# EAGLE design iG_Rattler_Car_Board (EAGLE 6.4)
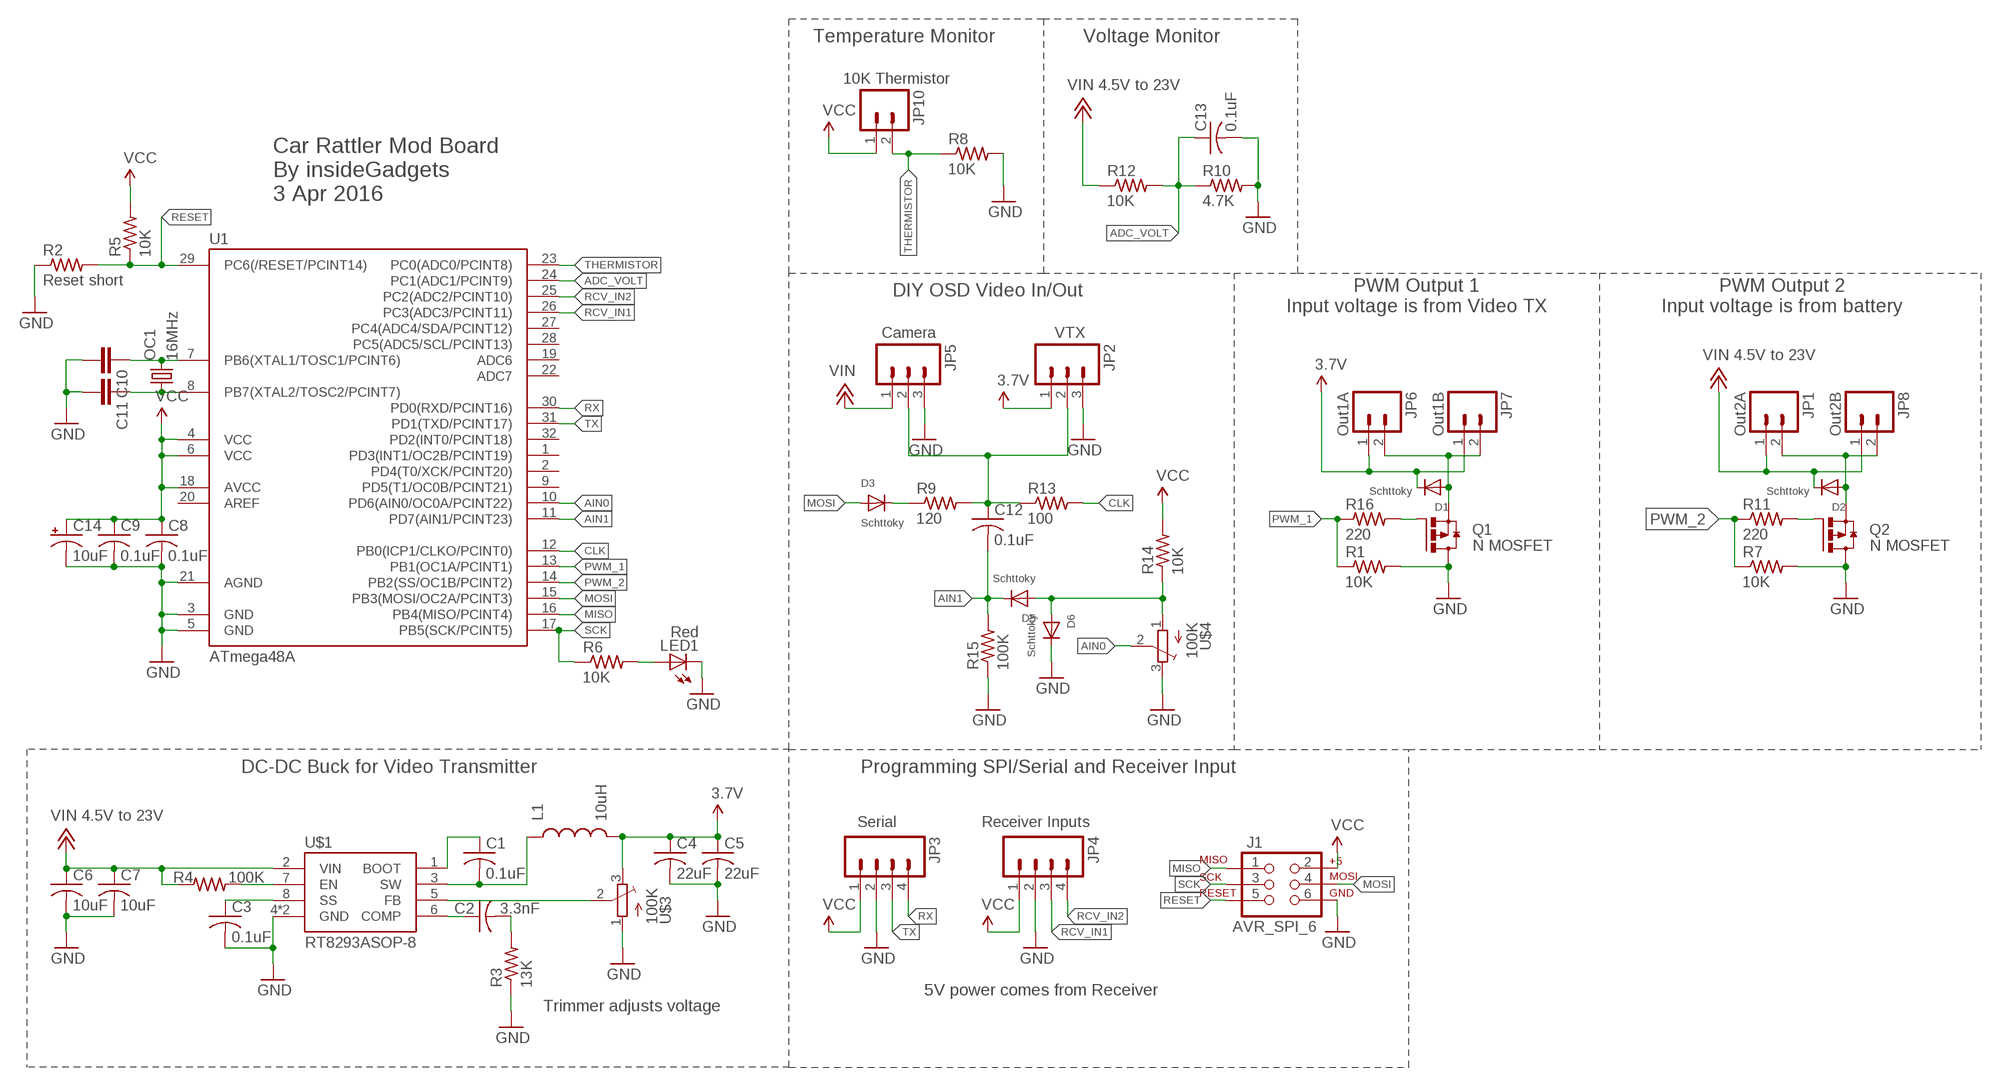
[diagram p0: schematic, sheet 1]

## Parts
C1  0.1uF  C-USC0603K  [C0603K]
C2  3.3nF  C-USC0603K  [C0603K]
C3  0.1uF  C-USC0603K  [C0603K]
C4  22uF  C-USC1206K  [C1206K]
C5  22uF  C-USC1206K  [C1206K]
C6  10uF  C-USC1206K  [C1206K]
C7  10uF  C-USC1206K  [C1206K]
C8  0.1uF  C-USC0805K  [C0805K]
C9  0.1uF  C-USC0805K  [C0805K]
C10  CAP0805  [0805]
C11  CAP0805  [0805]
C12  0.1uF  C-USC0805K  [C0805K]
C13  0.1uF  C-USC0805K  [C0805K]
C14  10uF  CPOL-US153CLV-0405  [153CLV-0405]
D1  Schttoky  DIODESOD-323  [SOD-323]
D2  Schttoky  DIODESOD-323  [SOD-323]
D3  Schttoky  DIODESOD-323  [SOD-323]
D5  Schttoky  DIODESOD-323  [SOD-323]
D6  Schttoky  DIODESOD-323  [SOD-323]
J1  AVR_SPI_6  AVR_SPI_PRG_6  [2X3_2]
JP1  Out2A  M02PTH  [1X02]
JP2  VTX  M03PTH  [1X03]
JP3  Serial  M04PTH  [1X04]
JP4  Receiver Inputs  M04PTH  [1X04]
JP5  Camera  M03PTH  [1X03]
JP6  Out1A  M02PTH  [1X02]
JP7  Out1B  M02PTH  [1X02]
JP8  Out2B  M02PTH  [1X02]
JP10  10K Thermistor  M02PTH  [1X02]
L1  10uH  INDUCTOR_7MM  [INDUCTOR7MM]
LED1  Red  LEDCHIP-LED0805-NS  [CHIP-LED0805-NS]
OC1  16MHz  XTAL-SMNOSILK  [XTAL32-25-NS]
Q1  N MOSFET  MOSFET_N_SMD_SOT23  [SUPER-SOT3]
Q2  N MOSFET  MOSFET_N_SMD_SOT23  [SUPER-SOT3]
R1  10K  R-US_R0805  [R0805]
R2  Reset short  R-US_R0805_2  [R0805_2]
R3  13K  R-US_R0603  [R0603]
R4  100K  R-US_R0603  [R0603]
R5  10K  R-US_R0805_2  [R0805_2]
R6  10K  R-US_R0805_2  [R0805_2]
R7  10K  R-US_R0805  [R0805]
R8  10K  R-US_R0805_2  [R0805_2]
R9  120  R-US_R0805_2  [R0805_2]
R10  4.7K  R-US_R0805_2  [R0805_2]
R11  220  R-US_R0805  [R0805]
R12  10K  R-US_R0805_2  [R0805_2]
R13  100  R-US_R0805_2  [R0805_2]
R14  10K  R-US_R0805_2  [R0805_2]
R15  100K  R-US_R0805_2  [R0805_2]
R16  220  R-US_R0805  [R0805]
U1  ATmega48A  MEGA48/88/168-AU  [TQFP32-08]
U$1  RT8293ASOP-8  [SOP-8]
U$3  100K  TRIMPOTTC33X  [TC33X]
U$4  100K  TRIMPOTTC33X  [TC33X]

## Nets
3.7V: C4.1 C5.1 D1.C JP2.1 JP6.1 JP7.1 L1.2 U$3.3(E)
5V: C8.1 C9.1 C14.+ J1.2 JP3.1 JP4.1 JP10.1 R5.2 R14.2 U1.4(VCC) U1.6(VCC) U1.18(AVCC) ; supply symbol labelled VCC
+12V: C6.1 C7.1 D2.C JP1.1 JP5.1 JP8.1 R4.1 R12.1 U$1.2(VIN) ; supply symbol labelled VIN 4.5V to 23V, VIN
ADC_VOLT: C13.1 R10.1 R12.2 U1.24(PC1(ADC1/PCINT9))
AIN0: U1.10(PD6(AIN0/OC0A/PCINT22)) U$4.2(S)
AIN1: C12.2 D5.C R15.2 U1.11(PD7(AIN1/PCINT23))
BOOT: C1.1 U$1.1(BOOT)
CLK: R13.2 U1.12(PB0(ICP1/CLKO/PCINT0))
COMP: C2.1 U$1.6(COMP)
EN: R4.2 U$1.7(EN)
FB: U$1.5(FB) U$3.2(S)
GND: C3.2 C4.2 C5.2 C6.2 C7.2 C8.2 C9.2 C10.2 C11.2 C13.2 C14.- D6.C J1.6 JP2.3 JP3.2 JP4.2 JP5.3 LED1.C Q1.2(D) Q2.2(D) R1.2 R2.1 R3.1 R7.2 R8.2 R10.2 R15.1 U1.3(GND) U1.5(GND) U1.21(AGND) U$1.4(GND) U$1.9(GND) U$3.1(A) U$4.3(E)
MISO: J1.1 U1.16(PB4(MISO/PCINT4))
MOSI: D3.A J1.4 U1.15(PB3(MOSI/OC2A/PCINT3))
N$1: C2.2 R3.2
N$3: D1.A JP6.2 JP7.2 Q1.3(S)
N$8: Q1.1(G) R16.2
N$10: LED1.A R6.2
N$13: D3.C R9.1
N$14: C11.1 OC1.1 U1.8(PB7(XTAL2/TOSC2/PCINT7))
N$15: C10.1 OC1.2 U1.7(PB6(XTAL1/TOSC1/PCINT6))
N$18: D5.A D6.A R14.1 U$4.1(A)
N$22: D2.A JP1.2 JP8.2 Q2.3(S)
N$27: Q2.1(G) R11.2
PWM_1: R1.1 R16.1 U1.13(PB1(OC1A/PCINT1))
PWM_2: R7.1 R11.1 U1.14(PB2(SS/OC1B/PCINT2))
RCV_IN1: JP4.3 U1.26(PC3(ADC3/PCINT11))
RCV_IN2: JP4.4 U1.25(PC2(ADC2/PCINT10))
RESET: J1.5 R2.2 R5.1 U1.29(PC6(/RESET/PCINT14))
RX: JP3.4 U1.30(PD0(RXD/PCINT16))
SCK: J1.3 R6.1 U1.17(PB5(SCK/PCINT5))
SS: C3.1 U$1.8(SS)
SW: C1.2 L1.1 U$1.3(SW)
THERMISTOR: JP10.2 R8.1 U1.23(PC0(ADC0/PCINT8))
TX: JP3.3 U1.31(PD1(TXD/PCINT17))
VIDEO: C12.1 JP2.2 JP5.2 R9.2 R13.1
Unconnected: U1.1(PD3(INT1/OC2B/PCINT19)) U1.2(PD4(T0/XCK/PCINT20)) U1.9(PD5(T1/OC0B/PCINT21)) U1.19(ADC6) U1.20(AREF) U1.22(ADC7) U1.27(PC4(ADC4/SDA/PCINT12)) U1.28(PC5(ADC5/SCL/PCINT13)) U1.32(PD2(INT0/PCINT18))

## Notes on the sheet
- Temperature Monitor | Voltage Monitor
- Car Rattler Mod Board
  By insideGadgets
  3 Apr 2016
- DIY OSD Video In/Out
- PWM Output 1
  Input voltage is from Video TX
- PWM Output 2
  Input voltage is from battery
- DC-DC Buck for Video Transmitter | Programming SPI/Serial and Receiver Input
- 5V power comes from Receiver
- Trimmer adjusts voltage

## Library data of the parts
C1-C9 C12 C13 = adafruit:C-US: CAPACITOR, American symbol
C10 C11 = SparkFun:CAP: Capacitor
C14 = rcl:CPOL-US: POLARIZED CAPACITOR, American symbol
D1-D3 D5 D6 = adafruit:DIODE: Diode
J1 = SparkFun:AVR_SPI_PRG_6: AVR ISP 6 Pin This is the reduced ISP connector for AVR programming. Common on Arduino. This footprint will take up less PCB space and can be used with a 10-pin to 6-pin adapter such as SKU: BOB-08508
JP1 JP6-JP8 JP10 = SparkFun:M02: Header 2
JP2 JP5 = SparkFun:M03: Header 3 Standard 3-pin 0.1" header. Use with straight break away headers (SKU : PRT-00116), right angle break away headers (PRT-00553), swiss pins (PRT-00743), machine pins (PRT-00117), and female headers (PRT-00115). Molex polarized connector foot print use with SKU : PRT-08232 with associated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
JP3 JP4 = SparkFun:M04: Header 4 Standard 4-pin 0.1" header. Use with straight break away headers (SKU : PRT-00116), right angle break away headers (PRT-00553), swiss pins (PRT-00743), machine pins (PRT-00117), and female headers (PRT-00115). Molex polarized connector foot print use with SKU : PRT-08231 with associated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
L1 = SparkFun:INDUCTOR_7MM
LED1 = adafruit:LED: LED
OC1 = adafruit:XTAL-SM
Q1 Q2 = transistor-power:MOSFET_N_SMD_SOT23
R1-R16 = adafruit:R-US_: RESISTOR, American symbol
U1 = avr-5:MEGA48/88/168
U$1 = alex:RT8293A
U$3 U$4 = adafruit:TRIMPOT: SMT trimmer potentiometer part number TC33X http://www.ladyada.net/library/eagle

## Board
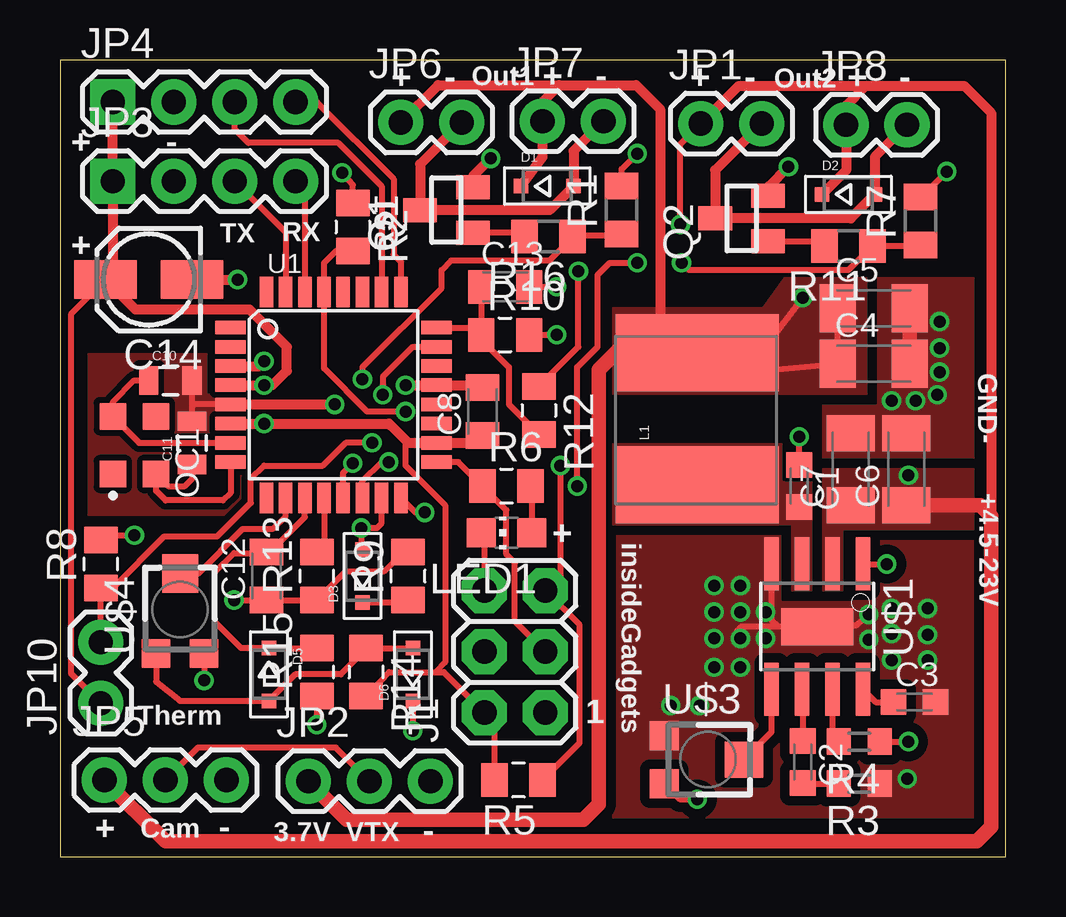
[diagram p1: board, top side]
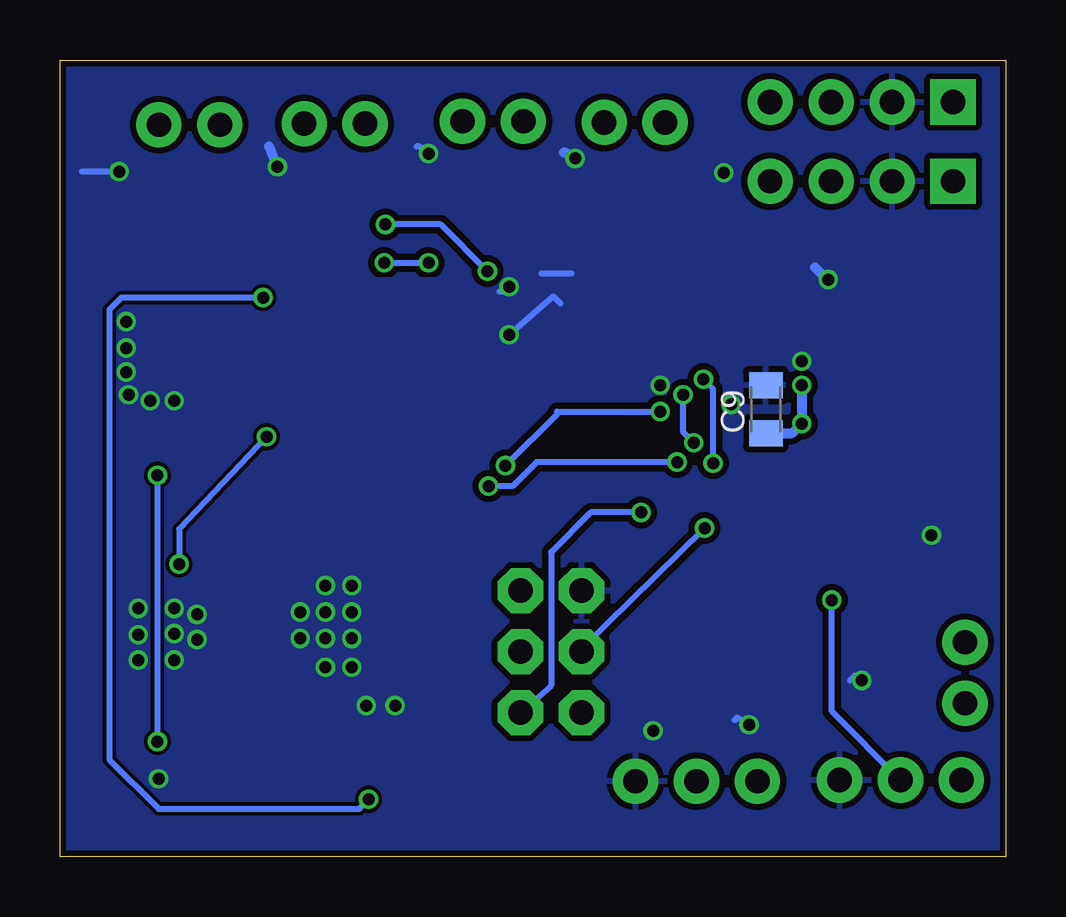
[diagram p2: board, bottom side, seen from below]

Size 39.4 x 33.2 mm. Coordinates in mm from the lower left corner, seen from the top.
Outline: 39.4,33.2 0,33.2 0,0 39.4,0 39.4,33.2
Copper layers (1*16): Top 0.035mm / dielectric 1.5mm / Bottom 0.035mm
Design rules "ITead_rule": minimum track width 6mil, minimum drill 12mil, track to track 6mil, track to pad 6mil, pad to pad 6mil, via to via 6mil, smd to smd 0mil, copper to edge 10mil, drill to drill 10mil, minimum pad ring 10mil, minimum via ring 6mil, stop-mask expansion 2mil, vias tented up to drill 100mil, thermal gap 10mil

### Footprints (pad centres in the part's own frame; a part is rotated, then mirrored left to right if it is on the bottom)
C0603K = smd 1.05 x 1.08: 1 -0.875,0; 2 0.875,0
C1206K = smd 1.5 x 2: 1 -1.5,0; 2 1.5,0
C0805K = smd 1.1 x 1.4: 1 -1,0; 2 1,0
0805 = smd 0.8 x 1.2: 1 -0.9,0; 2 0.9,0
153CLV-0405 = smd 2.6 x 1.6: + 1.8,0; - -1.8,0
SOD-323 = smd 0.6 x 0.6: A 1.1,0; C -1.1,0
2X3_2 = drill 1.016 pad 1.88 octagon: 1 -2.54,-1.27; 2 -2.54,1.27; 3 0,-1.27; 4 0,1.27; 5 2.54,-1.27; 6 2.54,1.27
1X02 = drill 1.016 pad 1.88: 1 0,0; 2 2.54,0
1X03 = drill 1.016 pad 1.88: 1 0,0; 2 2.54,0; 3 5.08,0
1X04 = drill 1.016 pad 1.88 square: 1 0,0 | drill 1.016 pad 1.88: 2 2.54,0; 3 5.08,0; 4 7.62,0
INDUCTOR7MM = smd 3.2 x 6.8: 1 -2.6,-0.2; 2 2.9,-0.2
CHIP-LED0805-NS = smd 1.2 x 1.2: A 0,-1.05; C 0,1.05
XTAL32-25-NS = smd 1.1 x 1.1: 1 -1.2,-0.9; 2 1.2,0.9; DNC -1.2,0.9; DNC2 1.2,-0.9
SUPER-SOT3 = smd 1 x 1.4: 1 -0.95,-1.1; 2 0.95,-1.1; 3 0,1.1
R0805 = smd 1.1 x 1.4: 1 -1,0; 2 1,0
R0805_2 = smd 1.1 x 1.4: 1 -1,0; 2 1,0
R0603 = smd 1 x 1.1: 1 -0.85,0; 2 0.85,0
TQFP32-08 = smd 1.27 x 0.559: 1 -4.293,2.8; 2 -4.293,2; 3 -4.293,1.2; 4 -4.293,0.4; 5 -4.293,-0.4; 6 -4.293,-1.2; 7 -4.293,-2; 8 -4.293,-2.8; 17 4.293,-2.8; 18 4.293,-2; 19 4.293,-1.2; 20 4.293,-0.4; 21 4.293,0.4; 22 4.293,1.2; 23 4.293,2; 24 4.293,2.8 | smd 0.559 x 1.27: 9 -2.8,-4.293; 10 -2,-4.293; 11 -1.2,-4.293; 12 -0.4,-4.293; 13 0.4,-4.293; 14 1.2,-4.293; 15 2,-4.293; 16 2.8,-4.293; 25 2.8,4.293; 26 2,4.293; 27 1.2,4.293; 28 0.4,4.293; 29 -0.4,4.293; 30 -1.2,4.293; 31 -2,4.293; 32 -2.8,4.293
SOP-8 = smd 0.61 x 2.21: 1 -1.905,-2.616; 2 -0.635,-2.616; 3 0.635,-2.616; 4 1.905,-2.616; 5 1.905,2.616; 6 0.635,2.616; 7 -0.635,2.616; 8 -1.905,2.616 | smd 3 x 1.55: 9 -0.01,0.02
TC33X = smd 1.2 x 1.2: 1 -1,-1.825; 3 1,-1.825 | smd 1.5 x 1.6: 2 0,1.5

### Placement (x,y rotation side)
C1  30.8,15.45 270 top
C2  30.95,3.95 270 top
C3  35.6,6.45 0 top
C4  33.9,20.55 0 top
C5  33.9,22.85 0 top
C6  35.25,16.15 90 top
C7  32.95,16.15 90 top
C8  17.6,18.55 90 top
C9  10,18.65 90 bottom
C10  4.6,19.85 0 top
C11  5.5,17.25 90 top
C12  8.6,11.7 90 top
C13  18.55,23.75 0 top
C14  3.7,24.05 180 top
D1  20.3,27.95 0 top
D2  32.85,27.6 0 top
D3  12.6,11.7 90 top
D5  8.7,7.6 270 top
D6  14.7,7.6 90 top
J1  18.95,8.55 90 top
JP1  26.7,30.55 0 top
JP2  10.35,3.15 0 top
JP3  2.2,28.15 0 top
JP4  2.2,31.45 0 top
JP5  1.85,3.2 0 top
JP6  14.2,30.6 0 top
JP7  20.1,30.65 0 top
JP8  32.75,30.5 0 top
JP10  1.7,6.4 90 top
L1  26.35,18.1 90 top
LED1  18.6,13.5 90 top
OC1  3.1,17.15 90 top
Q1  16.1,26.95 90 top
Q2  28.4,26.6 90 top
R1  23.4,26.95 90 top
R2  12.2,26.25 270 top
R3  33.3,3.05 180 top
R4  33.3,4.8 180 top
R5  19.1,3.2 180 top
R6  18.6,15.45 0 top
R7  35.85,26.5 90 top
R8  1.7,12.2 90 top
R9  14.5,11.7 90 top
R10  18.55,21.75 0 top
R11  32.85,25.45 180 top
R12  19.95,18.6 270 top
R13  10.7,11.7 90 top
R14  12.75,7.7 270 top
R15  10.7,7.7 90 top
R16  20.35,25.85 180 top
U1  11.4,19.25 0 top
U$1  31.55,9.6 180 top
U$3  27,4.05 270 top
U$4  5,10.3 0 top

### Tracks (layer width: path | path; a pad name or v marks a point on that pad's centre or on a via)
3.7V  (via drill 0.5)
  Top 0.254: 28.15,20.15 28.55,20.19 | 28.55,20.19 C4.1 C5.1 | v30.95,23.3 28.7,20.34 28.55,20.19 | U$3.3 25.82,2.4 v26.55,2.4
  Top 0.406: D1.C 20.1,29.15 JP7.1 20.1,31.45 20.8,32.15 | 20.8,32.15 15.75,32.15 JP6.1 | 20.8,32.15 24,32.15 25,31.15 25,22.4 | 25,21.7 25,22.4 | 25,22.4 25.55,21.85 25.7,21.85 L1.2
  Top 0.61: JP2.1 11.95,1.55 21.8,1.55 22.45,2.2 22.45,20.3 23.85,21.7 25,21.7
  Bottom 0.254: v30.95,23.3 36.85,23.3 37.35,22.8 37.35,4.05 35.3,2 26.95,2 v26.55,2.4
  pour Top (isolate 0.1, no thermals): 33.6,24.1 33.6,19.3 23.05,19.3 23.05,22.85 29.3,22.85 30.2,24.1
5V  (via drill 0.5)
  Top 0.254: 15.65,7.7 13.7,7.7 R14.2 12.75,6.4 | 15.65,7.7 15.99,7.7 J1.2 18.1,5.59 R5.2 | 14.5,17.25 14.4,17.15 14.4,16.3 16.05,14.65 16.05,8.1 15.65,7.7 | 13.78,18.08 13.78,17.98 | JP10.1 0.45,7.65 0.45,22.6 C14.+
  Top 0.406: U1.6 v8.5,18.05 13.7,18.05 13.78,17.98 14.5,17.25 U1.18 17.8,17.25 C8.1 | U1.4 v8.5,19.65 8.85,19.65 9.45,20.25 9.45,21.25 7.9,22.8 3.15,22.8 C14.+ 2.2,23.55 2.35,23.55 2.2,23.7 JP3.1 JP4.1
  Bottom 0.406: v8.5,19.65 v8.5,18.05 8.9,17.65 C9.1
+12V  (via drill 0.5)
  Top 0.254: R4.1 v35.35,4.8 | 19.95,19.8 R12.1 21.6,21.25 v21.6,24.4 | 26.65,30.55 JP1.1 25.85,29.7 v25.85,26.35
  Top 0.406: JP1.1 28.25,32.1 33.55,32.1 | D2.C 32.75,28.6 JP8.1 32.75,31.3 33.55,32.1 | 38.8,13.15 38.8,31 37.7,32.1 33.55,32.1
  Top 0.61: JP5.1 4.4,0.65 38.2,0.65 38.8,1.25 38.8,13.15 38.8,14.2 38.35,14.65 C6.1
  Bottom 0.254: v35.35,15.9 v35.35,4.8 | v21.6,24.4 23.55,26.35 v25.85,26.35
  pour Top (isolate 0.1, no thermals): 38.05,16.15 38.05,13.65 31.8,13.65 31.8,16.15
  pour Top (no thermals): 32.6,14.65 32.6,11.1 31.8,11.1 31.8,14.65
ADC_VOLT
  Top 0.254: R10.1 17.55,21.55 18.7,20.4 18.7,18.85 R12.2 | C13.1 R10.1 | U1.24 17.25,22.05 R10.1
AIN0
  Top 0.254: U$4.2 5.75,11.8 7.6,13.65 8.85,13.65 9.4,14.2 U1.10
AIN1
  Top 0.254: 10.4,8.8 R15.2 D5.C 7.55,8.7 6.45,9.8 6.45,11.85 7.25,12.65 8.55,12.65 C12.2 8.6,12.6 8.3,12.3 8.35,12.3 10.2,14.15 U1.11
BOOT  (via drill 0.5)
  Top 0.254: C1.1 v30.8,17.5 | U$1.1 33.47,12.2 v34.45,12.2
  Bottom 0.254: v30.8,17.5 34.45,13.65 v34.45,12.2
CLK
  Top 0.254: U1.12 11,13 R13.2
COMP
  Top 0.254: U$1.6 30.95,6.95 C2.1
EN
  Top 0.254: U$1.7 32.19,5.07 arc90 R4.2
FB
  Top 0.254: U$1.5 29.64,5.2 U$3.2
GND  (via drill 0.5)
  Top 0.254: U1.5 5.6,18.85 | 5.6,18.85 5.5,18.85 C10.2 | C11.2 5.5,18.75 5.6,18.85 | D6.C v14.7,5.25 | U$1.4 29.64,9.86 29.9,9.6 | 29.9,9.6 32.15,9.6 32.2,9.65 33.2,9.65 v33.7,10.1 | 28.2,9.4 28.4,9.6 29.9,9.6 | 8.55,20.7 v8.5,20.65 | U$4.3 v6,7.35 | LED1.C 17.68,13.42 J1.6 | R10.2 v20.7,21.75 | C13.2 v20.7,23.75 | R7.2 35.9,27.5 v36.95,28.55 | R1.2 23.4,28.65 v24.05,29.3 | R8.2 1.75,13.15 2,13.4 v3.1,13.4 | R15.1 v10.7,5.5 | R2.1 12.2,28 v11.75,28.5
  Top 0.406: v14.4,19.65 U1.21 17.5,19.65 C8.2 | U1.3 8.3,20.45 v8.5,20.65 | U1.5 v11.45,18.85 | Q2.2 29.55,27.55 29.55,27.95 v30.35,28.75 | C14.- v7.4,24.05 | Q1.2 17.2,28.35 v17.95,29.1
  Top 0.61: C5.2 C4.2
  Bottom 0.254: v6,7.35 6.3,7.55 6.5,7.35 | 18.1,24.3 19.35,24.3 | v20.7,21.75 18.85,23.35 18.55,23.05 | v20.7,23.75 20.9,23.55 21.1,23.55 | v24.05,29.3 24.45,29.6 24.55,29.6 | v36.95,28.55 38.5,28.55 | v3.1,13.4 2.95,13.35 3.35,13.35 | v10.7,5.5 11.2,5.8 11.3,5.7 | v11.75,28.5 11.85,28.75
  Bottom 0.406: v17.95,29.1 18.4,29.35 | v30.35,28.75 30.7,29.6 | v7.4,24.05 7.45,24.05 7.95,24.55
  other vias: 36.65,22.3 36.55,19.25 35.65,19 36.65,20.2 34.65,19 36.65,21.2 33.7,9.05 29.4,10.2 29.4,9.1 34.65,10.35 34.65,9.3 34.65,8.2 36.15,10.35 28.35,10.2 28.35,9.1 28.35,11.3 36.15,9.25 36.15,8.2 27.25,10.2 27.25,9.1 27.25,11.3 35.3,3.25 26.65,6.3 25.45,6.3 28.35,7.9 27.25,7.9
  pour Top (isolate 0.406, rank 6, no thermals): 38.05,24.1 38.05,1.65 23.05,1.65 23.05,18.3 31.8,16.85 31.8,24.1
  pour Top (isolate 0.254, no thermals): 1.2,20.95 6.1,20.95 6.1,19.25 7.7,19.25 7.7,14.25 1.2,14.25
  pour Bottom (isolate 0.254): 0.25,33.15 39.2,33.15 39.2,0.2 0.25,0.2 0.25,13.85 6.55,13.85 6.55,21.3 0.25,21.25
  pour Bottom (isolate 0.1): 38.05,24.1 38.05,1.65 23.05,1.65 23.05,24.1
  pour Bottom: 0.25,21.55 6.8,21.55 6.8,13.5 0.25,13.5
  pour Top (no thermals): 34.7,17.9 35.95,17.9 36,16.65 34.7,16.65
MISO  (via drill 0.5)
  Top 0.254: v15.2,14.35 14.81,14.35 U1.16
  Bottom 0.254: v15.2,14.35 17.3,14.35 18.95,12.7 18.95,7.13 J1.1
MOSI  (via drill 0.5)
  Top 0.254: U1.15 13.4,13.9 13.2,13.7 v12.55,13.7 12.55,12.85 12.6,12.85 D3.A
  Bottom 0.254: J1.4 17.68,8.67 v12.55,13.7
N$1
  Top 0.254: C2.2 30.98,3.05 R3.2
N$3
  Top 0.406: JP7.2 21.4,29.41 D1.A 20.4,26.95 Q1.3 15,28.86 JP6.2
N$8
  Top 0.254: R16.2 19.2,26 Q1.1
N$10
  Top 0.254: R6.2 19.65,15.45 LED1.A
N$13
  Top 0.254: D3.C 14.4,10.6 R9.1
N$14
  Top 0.254: U1.8 7.11,15.16 6.8,14.85 4.4,14.85 4,15.25 OC1.1 4.5,15.45 5.2,15.45 5.5,15.75 C11.1
N$15
  Top 0.254: U1.7 3.3,17.25 OC1.2 2.2,18.95 3.1,19.85 C10.1
N$18
  Top 0.254: D6.A R14.1 12.7,8.6 11.7,7.6 9.8,7.6 D5.A 5,6.5 4,7.3 U$4.1
N$22
  Top 0.406: JP8.2 33.95,29.16 D2.A 32.95,26.6 Q2.3 27.3,28.61 JP1.2
N$27
  Top 0.254: Q2.1 31.7,25.65 R11.2
PWM_1  (via drill 0.5)
  Top 0.254: R1.1 23.35,25.9 21.5,25.9 R16.1 21.35,25.8 20.4,24.85 16.3,24.85 15.9,24.45 15.9,23.7 12.6,20.4 v12.6,19.9 | U1.13 11.8,16 v12.2,16.4
  Bottom 0.254: v12.2,16.4 12.2,19.5 v12.6,19.9
PWM_2  (via drill 0.5)
  Top 0.254: U1.14 12.6,15.65 13.4,16.45 v13.7,16.45 | R7.1 35.8,25.45 R11.1 32.85,24.45 26.2,24.45 v25.9,24.75 | v21.55,15.45 21.55,20.4 22.4,21.25 22.4,24.25 22.9,24.75 v24.05,24.75
  Bottom 0.254: v13.7,16.45 19.55,16.45 20.55,15.45 v21.55,15.45 | v25.9,24.75 v24.05,24.75
RCV_IN1
  Top 0.254: JP4.3 7.28,30.32 7.85,29.75 11.6,29.75 13.4,27.95 U1.26
RCV_IN2
  Top 0.254: JP4.4 10.7,31.45 13.9,28.25 13.9,25.1 14.2,24.8 U1.25
RESET  (via drill 0.5)
  Top 0.254: v20.85,16.3 20.85,11.72 J1.5 21.65,9.66 21.65,4.75 R5.1 | v14.4,18.55 12.8,18.55 11,20.35 U1.29 11,24.75 11.5,25.25 R2.2
  Bottom 0.254: v14.4,18.55 18.7,18.55 18.7,18.45 v20.85,16.3
RX
  Top 0.254: JP3.4 10.2,27.77 U1.30
SCK
  Top 0.254: J1.3 18.95,9.82 18.95,12.25 18.6,12.6 18.6,14.45 R6.1 16.6,16.45 U1.17
SS
  Top 0.254: U$1.8 33.99,6.45 C3.1
SW
  pour Top (isolate 0.1, no thermals): 23.05,17.2 30.05,17.2 30.05,15.6 31.3,15.6 31.3,13.85 23.05,13.85
  pour Top (isolate 0.1, no thermals): 31.3,15.15 31.3,11.1 30.5,11.1 30.5,15.2
THERMISTOR  (via drill 0.5)
  Top 0.254: JP10.2 R8.1 2.2,11.2 4.35,13.35 6.55,13.35 7.95,14.75 7.95,15.75 8.5,16.3 10.95,16.3 11.9,17.25 v13,17.25 | U1.23 14.7,21.25 13.45,20 v13.45,19.25
  Bottom 0.254: v13.45,19.25 13.45,17.7 v13,17.25
TX
  Top 0.254: JP3.3 9.4,26.03 U1.31
VIDEO  (via drill 0.5)
  Top 0.254: R9.2 14.2,12.6 13.5,11.9 11.9,11.9 R13.1 C12.1 v7.25,10.7 | JP2.2 11.49,4.55 5.74,4.55 JP5.2
  Bottom 0.254: v7.25,10.7 7.25,6.06 JP5.2

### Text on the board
_tsilk: + | - | Out1 | + | - | + | - | Out2 | + | - | + | - | + | TX | RX | RST | GND- | +4.5-23V | + | insideGadgets | Therm | 1 | + | Cam | - | 3.7V | VTX | -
